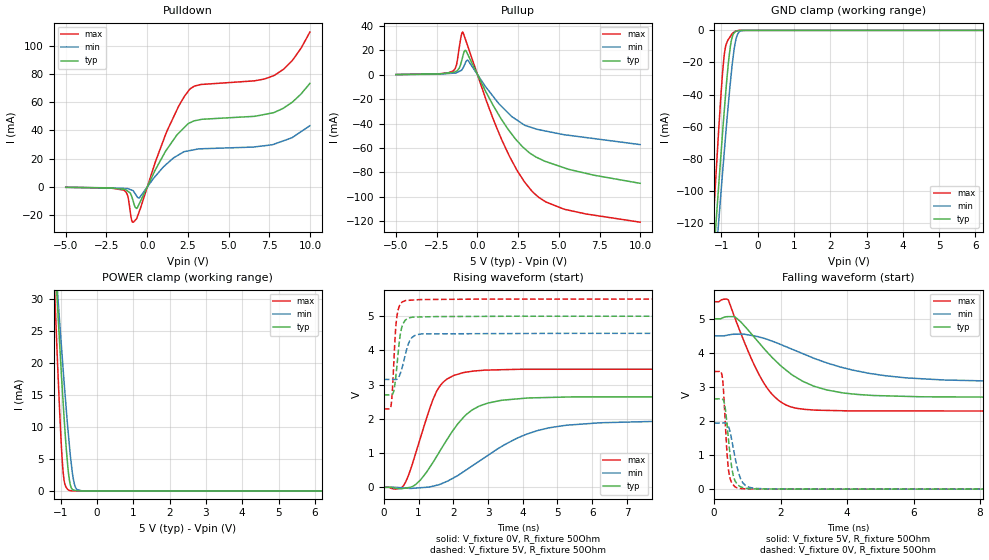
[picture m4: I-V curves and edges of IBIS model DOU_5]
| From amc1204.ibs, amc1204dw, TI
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|   5 V DOU Model
[Model] DOU_5
Model_type Output
Polarity   Non-Inverting
Enable   Active-Low
Vmeas = 2.5
Vref = 2.5
Cref = 15pF
Rref = 50
|   typ   min   max
|   (nom PVT)   (Fast PVT)   (slow PVT)
|   Output high
C_comp   1.22478E-12   9.80616E-13   1.49305E-12
|   Output low
|C_comp   1.36815E-12   1.08644E-12   1.66792E-12
|   High Impedance
|C_comp   1.24771E-12   9.63863E-13   1.54205E-12
| Where   nom PVT is  Nominal Process, 3.3V, 72C
|   Fast PVT is Strong Process, 3.6V, -40C
|   Slow PVT is Weak Process, 3.0V, 150C
|C_comp - from L-C Tank method, L = 1nH, peak frequency
| variable   typ   min   max
[Voltage Range]   5   4.5   5.5
[Temperature Range]   72   150   -40
|Operating Temperature   27   105   -40
[Pullup Reference]   5   4.5   5.5
[Pulldown Reference]   0   0   0
[Power Clamp Reference]   5   4.5   5.5
[GND Clamp Reference]   0   0   0
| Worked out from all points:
|   slope of the pulldown table from 0 to 0.75 V, typ, clamps not added: 43.2 ohm
|   slope of the pullup table from 0 to 0.75 V, typ, clamps not added: 37.4 ohm
|   GND clamp passes 1 mA (typ) near -0.62 V on its own axis
|   POWER clamp passes 1 mA (typ) near -0.74 V on its own axis
|   falling waveform, V_fixture 5V, R_fixture 50Ohm: 20-80 % time 1.54ns typ, 2.5ns min, 931ps max; typ from 5 V to 2.7 V
|   rising waveform, V_fixture 0V, R_fixture 50Ohm: 20-80 % time 1.08ns typ, 1.91ns min, 677ps max; typ from 0 V to 2.65 V
|   rising waveform, V_fixture 5V, R_fixture 50Ohm: 20-80 % time 150ps typ, 217ps min, 109ps max; typ from 2.7 V to 5 V
|   falling waveform, V_fixture 0V, R_fixture 50Ohm: 20-80 % time 183ps typ, 257ps min, 129ps max; typ from 2.65 V to 0 V
[Pulldown]
|   Voltage   I(typ)   I(min)   I(max)
-5V       -193.9uA   -134.8uA   -199.3uA
-1.441V   -1.564mA   -954.4uA   -2.178mA
-1.205V   -2.833mA   -1.087mA   -5.802mA
-963.2mV  -6.244mA   -2.103mA   -22.95mA
-850mV    -10.35mA   -2.746mA   -24.83mA
-598.1mV  -14.48mA   -7.235mA   -20.85mA
1.167V    25.97mA    16.02mA    38.29mA
1.927V    38.03mA    22.72mA    57.05mA
2.586V    45.2mA     25.7mA     68.76mA
7.749V    52.55mA    30.13mA    78.64mA
8.897V    59.9mA     34.91mA    89.32mA
9.985V    73.23mA    43.34mA    109.5mA
[GND Clamp]
|   Voltage   I(typ)   I(min)   I(max)
-5V       -1.447A    -1.346A    -1.7A
-1.256V   -155.5mA   -172.8mA   -132.2mA
-1.159V   -123.8mA   -144.1mA   -94.21mA
-1.074V   -96.88mA   -119.4mA   -62.28mA
-971.2mV  -65.1mA    -89.81mA   -27.68mA
-910.7mV  -47.46mA   -73.18mA   -13.62mA
-756mV    -10.62mA   -33.47mA   -3.922mA
-701.1mV  -4.192mA   -21.29mA   -2.094mA
-624.1mV  -1.049mA   -8.482mA   -613uA
-544.1mV  -214.1uA   -2.038mA   -192.9uA
-358.7mV  -20.44uA   -20.62uA   -37.38uA
9.985V    0A         0A         0A
[Pullup]
|   Voltage   I(typ)   I(min)   I(max)
-5V       259.8uA    205.4uA    285.6uA
-1.514V   2.064mA    1.354mA    3.043mA
-1.297V   3.067mA    1.707mA    7.771mA
-1.016V   9.378mA    3.553mA    31.08mA
-910.7mV  14.7mA     5.157mA    35.1mA
-738.2mV  20.09mA    9.999mA    29.09mA
-571.9mV  16.07mA    11.69mA    22.56mA
1.474V    -36.55mA   -25.83mA   -52.82mA
2.423V    -54mA      -37.11mA   -78.27mA
3.341V    -65.31mA   -43.31mA   -95.4mA
5.3V      -76.19mA   -49.07mA   -110.1mA
9.985V    -89.02mA   -57.21mA   -120.9mA
[POWER Clamp]
|   Voltage   I(typ)   I(min)   I(max)
-5V       474.9mA    380.3mA    630.3mA
-1.178V   38.24mA    38.32mA    32.55mA
-1.16V    36.29mA    36.77mA    29.94mA
-1.098V   29.75mA    31.77mA    21.2mA
-1.082V   28.2mA     30.54mA    19.12mA
-1.016V   21.46mA    25.22mA    10.58mA
-947.5mV  14.97mA    20mA       3.785mA
-885.1mV  9.45mA     15.34mA    1.026mA
-765.3mV  1.845mA    7.28mA     68.55uA
-624.7mV  118.7uA    1.067mA    4.622uA
-410.7mV  4.706uA    4.533uA    4.528uA
9.985V    0A         0A         0A
[Ramp]
R_load = 50
|   typ   min   max
dV/dt_r   1.58894/1.07624e-009   1.1636/1.90851e-009   2.07179/6.74193e-010
dV/dt_f   1.37989/1.53923e-009  0.808819/2.49143e-009   1.92529/9.31052e-010
[Falling Waveform]
V_fixture = 5V
V_fixture_min = 4.5V
V_fixture_max = 5.5V
R_fixture = 50Ohm
C_fixture = 0F
|   Time   V(typ)   V(min)   V(max)
0s        5V         4.5V       5.5V
426.8ps   5.063V     4.523V     5.554V
782.6ps   4.927V     4.549V     4.626V
1.502ns   4.123V     4.426V     3.106V
1.927ns   3.694V     4.276V     2.616V
2.437ns   3.3V       4.07V      2.383V
3.023ns   3.015V     3.833V     2.321V
3.827ns   2.833V     3.577V     2.302V
5.834ns   2.721V     3.262V     2.295V
15.93ns   2.7V       3.152V     2.291V
[Rising Waveform]
V_fixture = 0V
V_fixture_min = 0V
V_fixture_max = 0V
R_fixture = 50Ohm
C_fixture = 0F
|   Time   V(typ)   V(min)   V(max)
0s        2.93nV     6.623nV    2.49nV
575.4ps   -30.15mV   -18.01mV   61.15mV
931.1ps   92.93mV    -21.54mV   1.04V
1.517ns   896.4mV    58.65mV    2.798V
1.805ns   1.373V     168mV      3.153V
2.273ns   2.021V     441mV      3.347V
3.34ns    2.534V     1.162V     3.434V
4.113ns   2.607V     1.553V     3.449V
5.288ns   2.638V     1.817V     3.449V
15.93ns   2.648V     1.939V     3.453V
[Rising Waveform]
V_fixture = 5V
V_fixture_min = 4.5V
V_fixture_max = 5.5V
R_fixture = 50Ohm
C_fixture = 0F
|   Time   V(typ)   V(min)   V(max)
0s        2.7V       3.152V     2.291V
203.8ps   2.699V     3.15V      2.36V
289.5ps   2.828V     3.15V      3.674V
335.1ps   3.138V     3.149V     4.551V
375.7ps   3.53V      3.158V     4.983V
479.1ps   4.496V     3.338V     5.358V
631.9ps   4.894V     3.925V     5.457V
807.9ps   4.97V      4.374V     5.47V
1.102ns   4.978V     4.482V     5.486V
15.93ns   5V         4.5V       5.5V
[Falling Waveform]
|Gnd
V_fixture = 0V
V_fixture_min = 0V
V_fixture_max = 0V
R_fixture = 50Ohm
C_fixture = 0F
|   Time   V(typ)   V(min)   V(max)
0s        2.648V     1.939V     3.453V
234ps     2.654V     1.942V     3.36V
271.3ps   2.624V     1.942V     3.054V
327.2ps   2.43V      1.942V     2.114V
439.2ps   1.399V     1.823V     528.6mV
557ps     487.1mV    1.309V     149.7mV
721.3ps   118.2mV    536.4mV    22.09mV
948.1ps   24.33mV    105.9mV    9.55mV
1.6ns     5.784mV    8.154mV    4.495mV
15.93ns   156.1nV    839.3nV    64.97nV
